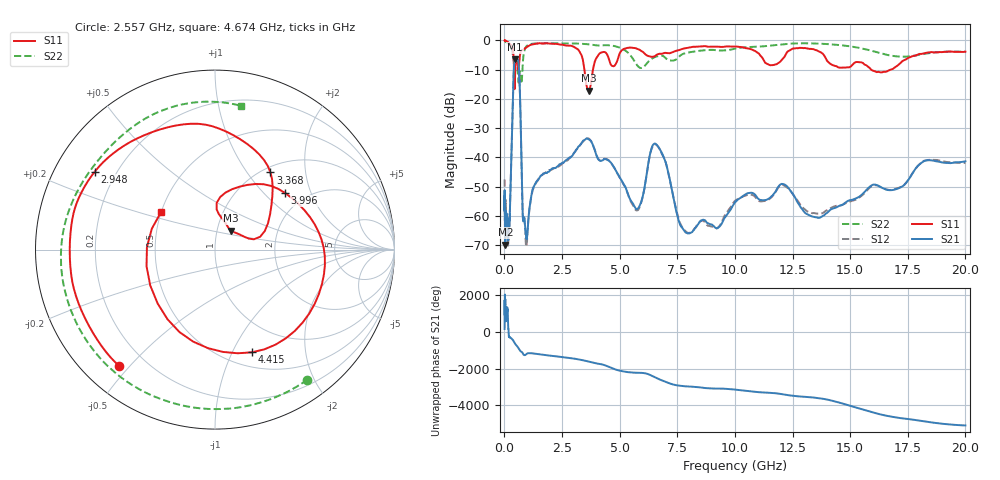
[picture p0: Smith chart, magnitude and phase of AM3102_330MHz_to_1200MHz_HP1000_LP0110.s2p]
! Date/Time: Tue, Sep 11, 2018 5:17 PM
! Network Analyzer: Agilent Technologies E8362B Rev: A.07.50.63
! Sweep from 0.010 to 20.000 GHz, 1601 Points, Sweep Type: LOG
! Power Supply: 4.949 V, 0.001 A
# Hz S DB R 50
!freq MagS11 AngS11 MagS21 AngS21 MagS12 AngS12 MagS22 AngS22
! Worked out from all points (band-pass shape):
!   1601 points, 10 MHz to 20 GHz, reference 50 ohm
!   highest |S21| = -6.45 dB at 460.1 MHz (marker M1); lowest = -69.8 dB at 41.78 MHz (marker M2)
!   |S21| within 3 dB of the highest: 412.9 MHz to 630.9 MHz (218 MHz wide, 41.8 % of centre)
!   lowest |S11| = -17.2 dB at 3.651 GHz (marker M3), VSWR 1.32, Z = 58.2 + j12.6 ohm
!   |S11| at or under -10 dB: 415.6 MHz to 468.4 MHz (52.74 MHz wide, 11.9 % of centre); 3.471 GHz to 3.843 GHz (371 MHz wide, 10.1 % of centre); 15.91 GHz to 16.77 GHz (851.5 MHz wide, 5.21 % of centre)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
!   |S22| runs from -14.8 to -0.2 dB; largest |S21 - S12| = 0.0079
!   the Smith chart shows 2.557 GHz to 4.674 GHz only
!   S11 on the Smith chart (normalised r, x): 2.557 GHz: 0.11, -0.47; 2.948 GHz: 0.12, +0.29; 3.368 GHz: 1.09, +1.30; 3.996 GHz: 1.59, +1.34; 4.415 GHz: 0.66, -1.19; 4.674 GHz: 0.50, +0.24
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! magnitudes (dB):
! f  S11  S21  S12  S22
! 10 MHz  0.0  -58.3  -47.6  -0.2
! 35.55 MHz  0.0  -64.2  -64.0  -0.3
! 41.78 MHz  0.0  -69.8  -65.5  -0.4
! 126.4 MHz  -0.4  -65.5  -63.5  -0.8
! 232.2 MHz  -1.1  -59.4  -59.9  -1.4
! 447.2 MHz  -16.2  -6.6  -6.6  -7.8
! 460.1 MHz  -12.4  -6.5  -6.5  -7.2
! 635.6 MHz  -8.6  -10.1  -10.1  -13.4
! 794.6 MHz  -3.3  -59.4  -59.4  -8.3
! 947.3 MHz  -2.4  -67.4  -70.2  -2.1
! 1.59 GHz  -1.1  -46.3  -46.2  -1.0
! 2.557 GHz  -1.5  -41.8  -41.9  -1.0
! 2.948 GHz  -2.0  -39.5  -39.3  -1.0
! 3.368 GHz  -5.5  -34.9  -35.0  -1.2
! 3.651 GHz  -17.2  -33.8  -33.6  -1.3
! 3.996 GHz  -6.0  -39.4  -39.2  -1.7
! 4.415 GHz  -4.3  -40.7  -40.5  -1.6
! 4.674 GHz  -8.7  -42.4  -42.4  -1.8
! 5.652 GHz  -2.6  -56.9  -57.5  -7.2
! 6.549 GHz  -5.3  -35.3  -35.5  -5.6
! 7.995 GHz  -2.4  -66.0  -65.9  -4.1
! 20 GHz  -3.8  -41.3  -41.9  -3.9
